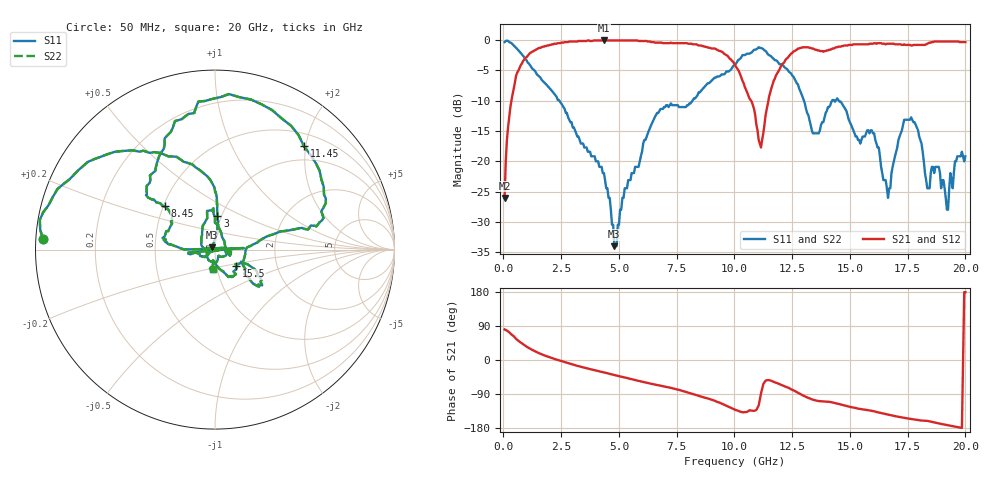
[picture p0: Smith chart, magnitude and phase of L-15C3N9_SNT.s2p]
# MHZ S MA R 50
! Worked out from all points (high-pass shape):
!   400 points, 50 MHz to 20 GHz, reference 50 ohm
!   highest |S21| = -0.09 dB at 4.35 GHz (marker M1); lowest = -26.0 dB at 50 MHz (marker M2)
!   |S21| within 3 dB of the highest: 927.3 MHz to 9.798 GHz (8.87 GHz wide, 165 % of centre); 12.25 GHz to end of sweep
!   lowest |S11| = -34.0 dB at 4.8 GHz (marker M3), VSWR 1.04, Z = 48.5 + j1.3 ohm
!   |S11| at or under -10 dB: 2.419 GHz to 8.181 GHz (5.763 GHz wide, 109 % of centre); 13.01 GHz to 14.23 GHz (1.222 GHz wide, 8.97 % of centre); 14.52 GHz to end of sweep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
!   |S22| runs from -34.0 to -0.1 dB; largest |S21 - S12| = 0
!   S11 on the Smith chart (normalised r, x): 50 MHz: 0.02, +0.03; 3 GHz: 0.95, +0.38; 8.45 GHz: 0.51, +0.28; 11.45 GHz: 0.72, +1.97; 15.5 GHz: 1.24, -0.23; 20 GHz: 0.95, -0.21
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50  0.96 176.5  0.05 80.6  0.05 80.6  0.96 176.5
600  0.84 143.1  0.54 52.9  0.54 52.9  0.84 143.1
3000  0.19 86.1  0.97 -11.9  0.97 -11.9  0.19 86.1
3400  0.14 83.6  0.98 -18.7  0.98 -18.7  0.14 83.6
4350  0.08 84.0  0.99 -32.5  0.99 -32.5  0.08 84.0
4800  0.02 137.9  0.99 -39.6  0.99 -39.6  0.02 137.9
6200  0.16 3.1  0.98 -60.0  0.98 -60.0  0.16 3.1
6700  0.25 173.3  0.95 -66.7  0.95 -66.7  0.25 173.3
8450  0.37 139.3  0.9 -94.5  0.9 -94.5  0.37 139.3
10050  0.63 116.9  0.61 -131.8  0.61 -131.8  0.63 116.9
11150  0.86 76.7  0.13 -88.6  0.13 -88.6  0.86 76.7
11450  0.76 49.3  0.3 -52.9  0.3 -52.9  0.76 49.3
13350  0.18 4.0  0.85 -103.8  0.85 -103.8  0.18 4.0
14450  0.33 -37.1  0.87 -115.2  0.87 -115.2  0.33 -37.1
15500  0.15 -37.9  0.92 -129.8  0.92 -129.8  0.15 -37.9
16700  0.06 10.2  0.93 -144.8  0.93 -144.8  0.06 10.2
17350  0.22 101.6  0.92 -152.8  0.92 -152.8  0.22 101.6
19200  0.04 -58.1  0.97 -171.8  0.97 -171.8  0.04 -58.1
19850  0.12 -100.7  0.96 -179.1  0.96 -179.1  0.12 -100.7
19900  0.11 -99.0  0.96 0.2  0.96 0.2  0.11 -99.0
19950  0.1 -97.4  0.96 179.4  0.96 179.4  0.1 -97.4
20000  0.11 -97.1  0.96 179.1  0.96 179.1  0.11 -97.1
